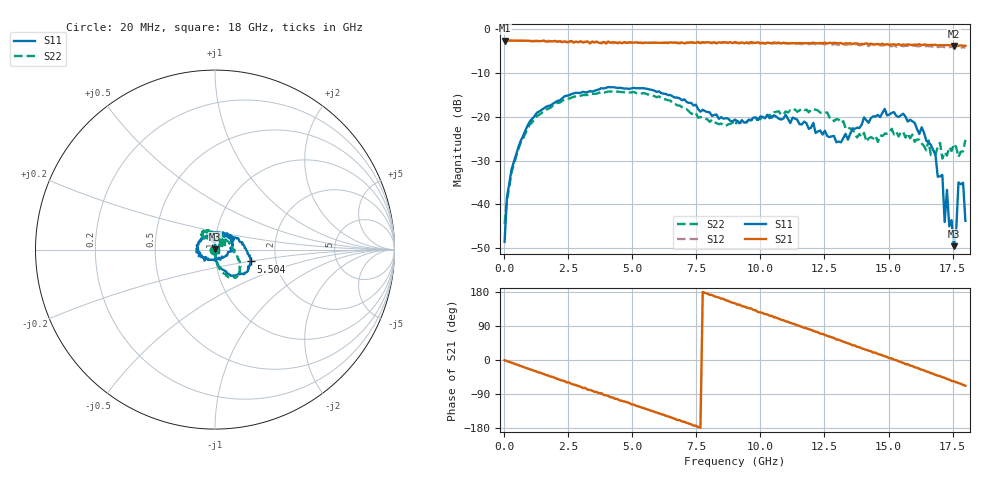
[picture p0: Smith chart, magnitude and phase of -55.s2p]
!Agilent Technologies,N5230A,US43500223,A.07.50.48
!Agilent N5230A: A.07.50.48
!Date: Tuesday, February 02, 2016 12:01:26
!Correction: S11(Full 2 Port(1,2))
!S21(Full 2 Port(1,2))
!S12(Full 2 Port(1,2))
!S22(Full 2 Port(1,2))
!S2P File: Measurements: S11, S21, S12, S22:
# Hz S  RI  R 50
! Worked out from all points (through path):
!   201 points, 20 MHz to 18 GHz, reference 50 ohm
!   highest |S21| = -2.59 dB at 20 MHz (marker M1); lowest = -3.8 dB at 17.55 GHz (marker M2)
!   group delay of S21, straight-line fit = 65.7 ps
!   lowest |S11| = -49.6 dB at 17.55 GHz (marker M3), VSWR 1.01, Z = 50.2 + j0.266 ohm
!   |S11| at or under -10 dB: start of sweep to end of sweep
!   |S22| runs from -44.4 to -14.2 dB; largest |S21 - S12| = 0.092
!   S11 on the Smith chart (normalised r, x): 20 MHz: 0.99, -0.00; 5.504 GHz: 1.48, -0.20; 18 GHz: 1.01, -0.01
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2e7  -0.00281 -0.00247  0.7418 -0.00684  0.7432 -0.00957  -0.00586 -0.00137
1.099e8  -0.00167 -0.0119  0.7407 -0.0352  0.7409 -0.0359  -0.00391 -0.0101
2.897e8  0.00218 -0.0249  0.7338 -0.0915  0.7348 -0.0931  -0.00153 -0.0231
9.19e8  0.0127 -0.0783  0.6844 -0.279  0.6805 -0.2845  0.0125 -0.0728
3.0766e9  0.135 -0.1372  0.1948 -0.6791  0.1878 -0.6897  0.0847 -0.1551
5.5039e9  0.1994 -0.066  -0.4343 -0.5515  -0.45 -0.5278  0.136 -0.125
6.0433e9  0.1924 -0.0324  -0.5426 -0.4431  -0.5583 -0.4209  0.143 -0.0933
9.01e9  -0.0289 0.0884  -0.6171 0.3608  -0.582 0.3824  0.0325 0.0728
1.20666e10  -0.0586 -0.0615  0.1556 0.6832  0.2119 0.6521  -0.071 0.0987
1.31454e10  0.0235 -0.0453  0.4412 0.54  0.46 0.4874  -0.0587 0.0617
1.50333e10  0.0828 0.0661  0.6594 0.0518  0.6417 -0.0123  0.0233 0.0616
1.66515e10  -0.0147 0.0455  0.5455 -0.3759  0.4775 -0.419  0.0267 0.0247
1.7101e10  -0.01 0.0192  0.4612 -0.4671  0.3885 -0.5018  0.0244 0.0227
1.71909e10  -0.000716 0.00623  0.4481 -0.4823  0.3647 -0.504  0.0257 0.0297
1.72808e10  0.000102 0.0146  0.4221 -0.504  0.3488 -0.5245  0.0316 0.0173
1.73707e10  0.00558 0.00039  0.4029 -0.5176  0.3197 -0.5356  0.04 0.0203
1.74606e10  0.00412 -0.00514  0.3728 -0.5367  0.2983 -0.554  0.0347 0.0212
1.75505e10  0.002 0.00265  0.3559 -0.5345  0.2717 -0.5482  0.0302 0.0382
1.76404e10  0.00297 -0.00402  0.3401 -0.56  0.27 -0.5652  0.0347 0.0286
1.77303e10  0.0177 -0.000862  0.314 -0.5647  0.2251 -0.576  0.0276 0.0211
1.79101e10  -0.00105 -0.0176  0.2654 -0.5892  0.1888 -0.5951  0.0286 0.0282
1.8e10  0.00447 -0.00468  0.243 -0.5989  0.1606 -0.5907  0.0367 0.0403
